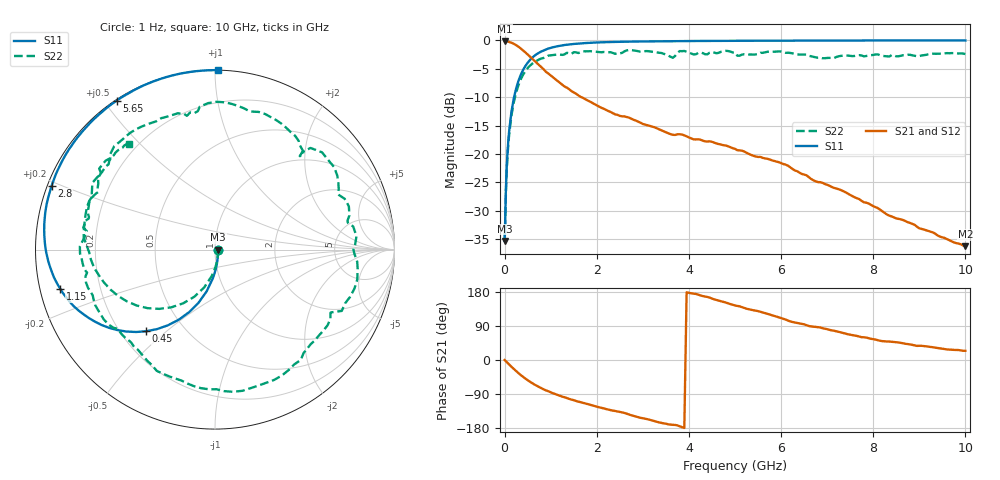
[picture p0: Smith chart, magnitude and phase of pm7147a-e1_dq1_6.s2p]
# GHz S DB R 50
! S-Parameters data
! Freq  dbS11  angS11  dbS21  angS21  dbS12  angS12  dbS22  angS22
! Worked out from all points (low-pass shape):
!   279 points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, 1 Hz to 10 GHz, reference 50 ohm
!   highest |S21| = -0.15 dB at 19.95 kHz (marker M1); lowest = -36.3 dB at 10 GHz (marker M2)
!   |S21| within 3 dB of the highest: start of sweep to 589.9 MHz
!   lowest |S11| = -35.4 dB at 15.85 kHz (marker M3), VSWR 1.03, Z = 51.7 - j0.00264 ohm
!   |S11| at or under -10 dB: start of sweep to 205.2 MHz
!   |S22| runs from -35.4 to -1.7 dB; largest |S21 - S12| = 0
!   S11 on the Smith chart (normalised r, x): 1 Hz: 1.03, -0.00; 450 MHz: 0.30, -0.43; 1.15 GHz: 0.06, -0.12; 2.8 GHz: 0.01, +0.19; 5.65 GHz: 0.00, +0.54; 10 GHz: 0.00, +1.02
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1e-09  -35.36 -0.0  -0.15 -0.0  -0.15 -0.0  -35.36 -0.0
1.58489e-05  -35.36 -0.1  -0.15 -0.0  -0.15 -0.0  -35.36 -0.1
1.99526e-05  -35.36 -0.1  -0.15 -0.0  -0.15 -0.0  -35.36 -0.1
0.03981072  -23.52 -79.1  -0.17 -4.8  -0.17 -4.8  -24.14 -79.3
0.1  -15.86 -94.3  -0.26 -12.1  -0.26 -12.1  -16.51 -97.2
0.25  -8.46 -112.5  -0.83 -29.2  -0.83 -29.2  -9.18 -120.6
0.45  -4.51 -130.1  -2.10 -49.0  -2.10 -49.0  -5.41 -144.5
0.75  -2.15 -149.1  -4.36 -71.4  -4.36 -71.4  -3.34 -171.4
1.15  -1.02 -165.7  -7.14 -92.3  -7.14 -92.3  -2.48 161.7
1.7  -0.49 179.1  -10.12 -112.9  -10.12 -112.9  -1.89 134.3
2.8  -0.20 158.7  -13.99 -147.6  -13.99 -147.6  -1.75 83.5
3.35  -0.14 150.6  -15.66 -164.6  -15.66 -164.6  -2.17 57.3
3.8  -0.11 144.5  -16.54 -174.9  -16.54 -174.9  -1.88 42.3
4.5  -0.09 136.0  -17.87 162.1  -17.87 162.1  -2.03 5.4
4.8  -0.07 132.5  -18.52 151.6  -18.52 151.6  -1.83 -11.9
5.05  -0.07 129.8  -19.35 142.9  -19.35 142.9  -2.69 -28.5
5.65  -0.05 123.5  -20.79 123.9  -20.79 123.9  -2.09 -58.5
6  -0.04 120.0  -21.63 110.5  -21.63 110.5  -1.96 -82.8
6.7  -0.02 113.5  -24.65 88.1  -24.65 88.1  -2.89 -123.5
7.7  -0.01 105.1  -27.99 61.7  -27.99 61.7  -2.59 -165.7
8.35  -0.01 100.1  -30.89 48.7  -30.89 48.7  -2.83 171.8
10  -0.00 89.1  -36.27 24.3  -36.27 24.3  -2.40 129.1
